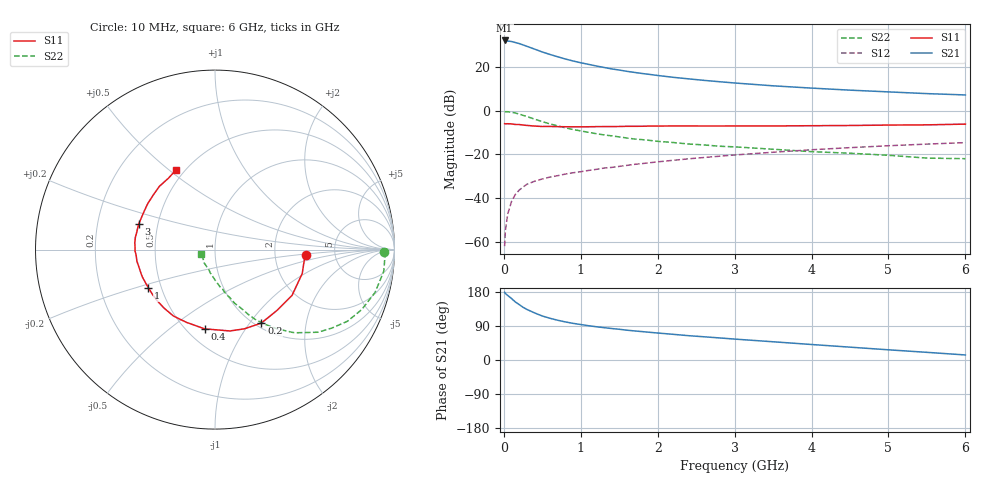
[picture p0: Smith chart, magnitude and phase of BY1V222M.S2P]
! SIEMENS Small Signal Semiconductors
! BFY420
! Si NPN RF SIEGET Grounded Emitter Transistor in MICRO-X
! VCE = 1.25 V  IC = 22 mA
! Common Emitter S-Parameters:  October  1996
# GHz  S  MA  R  50
!  f  S11  S21  S12  S22
! GHz  MAG  ANG  MAG  ANG  MAG  ANG  MAG  ANG
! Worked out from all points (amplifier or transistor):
!   36 points, 10 MHz to 6 GHz, reference 50 ohm
!   highest |S21| = 32.1 dB at 10 MHz (marker M1)
!   |S21| within 3 dB of that: start of sweep to 324.5 MHz
!   unconditionally stable (mu >= 1): start of sweep to 10.27 MHz; 1.745 GHz to end of sweep
!   at 250 MHz: K = 0.32, MSG = 32.5 dB, |S12| = -34.9 dB
!   at 1.4 GHz: K = 0.95, MSG = 22.5 dB, |S12| = -25.9 dB
!   at 6 GHz: K = 1.09, MAG = 9.1 dB, |S12| = -14.6 dB
!   S11 on the Smith chart (normalised r, x): 10 MHz: 3.02, -0.26; 200 MHz: 1.07, -1.14; 400 MHz: 0.61, -0.67; 1 GHz: 0.42, -0.22; 3 GHz: 0.39, +0.14; 6 GHz: 0.45, +0.53
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0.01  0.5055 -3.7  40.37 178.7  0.0008 116.7  0.9441 -0.8
0.02  0.5011 -6.4  40.14 175.6  0.0018 94.1  0.9476 -2.4
0.1  0.4993 -30.7  38.19 162.2  0.0084 77.7  0.9232 -15.0
0.15  0.4838 -44.5  36.15 153.0  0.0122 72.2  0.8833 -22.2
0.2  0.484 -57.7  34.26 146.2  0.0153 68.8  0.8392 -28.4
0.25  0.4707 -69.6  31.91 139.1  0.018 64.7  0.7839 -33.9
0.3  0.4609 -79.6  29.62 133.4  0.0208 63.7  0.7363 -38.7
0.4  0.4453 -97.5  25.58 124.2  0.0244 59.3  0.6412 -46.3
0.5  0.4354 -111.6  22 116.1  0.0275 57.8  0.5615 -51.9
0.6  0.4365 -122.1  19.31 110.1  0.0304 56.7  0.4995 -56.3
0.7  0.4322 -131.2  17.1 104.9  0.0327 55.8  0.4496 -60.0
0.8  0.4298 -138.6  15.21 100.5  0.0356 55.2  0.4066 -62.8
1  0.428 -150.0  12.47 93.6  0.0403 55.5  0.3449 -67.1
1.1  0.4293 -155.2  11.47 90.5  0.0431 55.9  0.3206 -69.7
1.4  0.4341 -165.9  9.037 83.1  0.0505 56.2  0.2662 -74.6
1.6  0.44 -171.5  7.947 78.7  0.0563 55.6  0.2376 -77.9
2.2  0.4485 175.0  5.805 67.8  0.0734 53.9  0.1875 -86.1
3  0.4479 161.3  4.303 55.2  0.0973 49.7  0.1491 -95.2
3.5  0.4481 153.1  3.706 48.1  0.1123 46.2  0.1315 -101.9
4.5  0.4592 138.5  2.951 33.9  0.143 37.7  0.1067 -115.1
5.5  0.475 123.0  2.459 20.2  0.1725 28.0  0.0826 -144.0
6  0.4937 116.2  2.293 13.3  0.1864 22.9  0.0799 -164.2
